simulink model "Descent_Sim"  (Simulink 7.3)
settings: Solver=ode45  StartTime=0.0  StopTime=900  RelTol=1e-3
InitFcn:
  | init
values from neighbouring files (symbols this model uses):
  h0 = 76068    [init.m]
  mass = 450    [init.m]
  sp = 30.81    [init.m]
  x0 = 0    [init.m]
  x_cg = 31.56    [init.m]
  x_ref = 31.5    [init.m]
  y_cg = 0    [init.m]
  z_cg = 1.24    [init.m]
undefined symbols (not defined in the file or in its folder): Altitude2, Cl, Cld1, Cld2, Cld3, Cld4, Cm, Cmd1, Cmd2, Cmd3, Cmd4, Cn, Cnd1, Cnd2, Cnd3, Cnd4, Continuous, CX, CXd1, CXd2, CXd3, CXd4, CY, CYd1, CYd2, CYd3, CYd4, CZ, CZd1, CZd2, CZd3, CZd4, Dryden, F, FCS, ft, km, Light, MIL, q, r, sigbuilder_block, Surf_mix
libraries: aerolibasang x3, aerolibwind2 x3, aerolib6dof2 x1, aerolibconvert2 x1, aerolibatmos2 x1, aerolibgravity2 x1, aerolibadyn x1

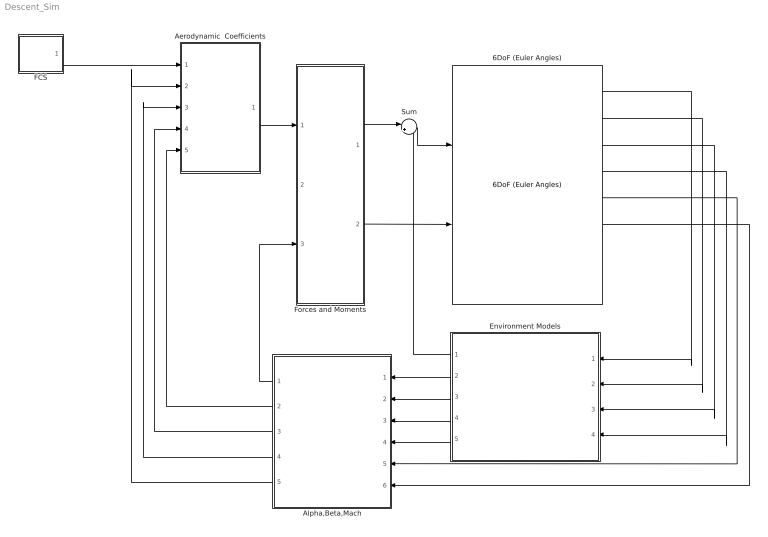
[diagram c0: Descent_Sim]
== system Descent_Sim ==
  6DoF (Euler Angles) : aerolib6dof2/6DoF (Euler Angles)  SystemSampleTime=-1  units=English (Velocity in ft/s)  mtype=Fixed  rep=Euler Angles  xme_0=[-x0, 0, -h0]  Vm_0=Uvw_0  eul_0=Euler_0  pm_0=pqr_0  mass_0=mass  mass_e=0.5  mass_f=2.0  inertia=inertia  inertia_e=eye(3)  inertia_f=2*eye(3)  k_quat=1.0
  Aerodynamic  Coefficients : Subsystem
  Alpha,Beta,Mach : Subsystem
  Environment Models : Subsystem
  FCS : Subsystem
  Forces and Moments : Subsystem
  Sum : Sum  Inputs=|++  OutDataType=sfix(16)  OutScaling=2^0
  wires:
  6DoF (Euler Angles)/5 -> Alpha,Beta,Mach/5(Vb)
  6DoF (Euler Angles)/1 -> Environment Models/1(Ve)
  6DoF (Euler Angles)/2 -> Environment Models/2(Xe)
  6DoF (Euler Angles)/3 -> Environment Models/3(Euler)
  6DoF (Euler Angles)/4 -> Environment Models/4(DCM)
  Sum/1 -> 6DoF (Euler Angles)/1
  Forces and Moments/1(X,Y,Z) -> Sum/1
  Environment Models/2(Speed of Sound) -> Alpha,Beta,Mach/1(Speed of Sound)
  Environment Models/3(Wind Velocity) -> Alpha,Beta,Mach/2(Wind Velocity)
  Environment Models/4(Air Density) -> Alpha,Beta,Mach/3(Air Density)
  Environment Models/5(Wind Angular Rates) -> Alpha,Beta,Mach/4(Wind Angular Rates)
  Environment Models/1(Fg) -> Sum/2
  Alpha,Beta,Mach/1(qbar) -> Forces and Moments/3(qbar)
  Alpha,Beta,Mach/3(V) -> Aerodynamic  Coefficients/4(V)
  Alpha,Beta,Mach/5(Incid) -> Aerodynamic  Coefficients/2(Incid)
  Alpha,Beta,Mach/4(Mach) -> Aerodynamic  Coefficients/3(Mach)
  Alpha,Beta,Mach/2("p,q,r ") -> Aerodynamic  Coefficients/5(p,q,r)
  6DoF (Euler Angles)/6 -> Alpha,Beta,Mach/6(p,q,r)
  Aerodynamic  Coefficients/1(Coeff) -> Forces and Moments/1(Coeff)
  Forces and Moments/2(LMN) -> 6DoF (Euler Angles)/2
  FCS/1(delta) -> Aerodynamic  Coefficients/1(deltas)

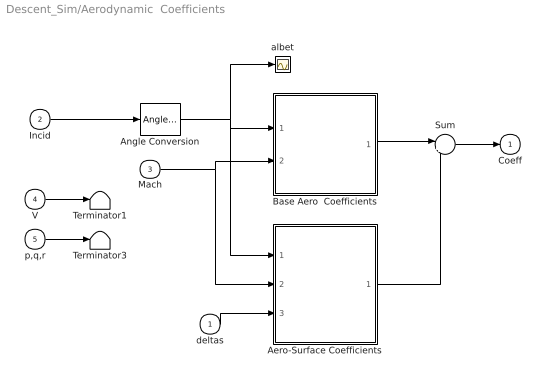
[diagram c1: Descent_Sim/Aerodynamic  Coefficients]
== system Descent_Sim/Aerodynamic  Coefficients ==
  deltas : Inport  OutDataType=sfix(16)  OutScaling=2^0
  Incid : Inport  Port=2  OutDataType=sfix(16)  OutScaling=2^0
  Mach : Inport  Port=3  OutDataType=sfix(16)  OutScaling=2^0
  V : Inport  Port=4  OutDataType=sfix(16)  OutScaling=2^0
  p,q,r : Inport  Port=5  OutDataType=sfix(16)  OutScaling=2^0
  Aero-Surface Coefficients : Subsystem
  Angle Conversion : aerolibconvert2/Angle Conversion  SystemSampleTime=-1  IU=rad  OU=deg
  Base Aero  Coefficients : Subsystem
  Sum : Sum  Inputs=|++  OutDataType=fixdt(1, 16)  OutScaling=2^0
  Terminator1 : Terminator
  Terminator3 : Terminator
  albet : Scope
  Coeff : Outport  OutDataType=sfix(16)  OutScaling=2^0  InitialOutput=0
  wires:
  p,q,r/1 -> Terminator3/1
  V/1 -> Terminator1/1
  Incid/1 -> Angle Conversion/1
  Angle Conversion/1 -> albet/1, Base Aero  Coefficients/1(albet), Aero-Surface Coefficients/1(albet)
  Mach/1 -> Base Aero  Coefficients/2(Mach), Aero-Surface Coefficients/2(Mach)
  Sum/1 -> Coeff/1
  Base Aero  Coefficients/1(Coeff) -> Sum/1
  Aero-Surface Coefficients/1(Coeff) -> Sum/2
  deltas/1 -> Aero-Surface Coefficients/3(delta)

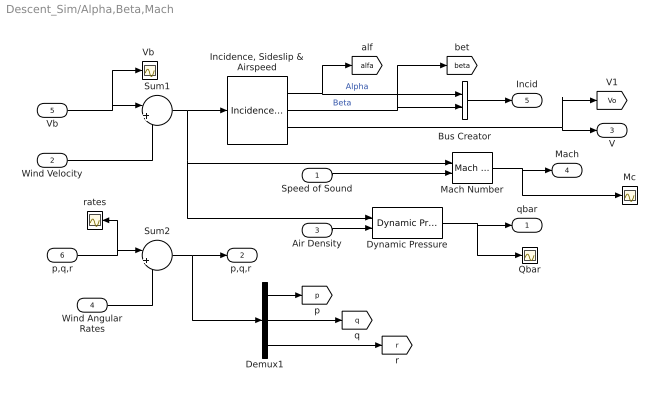
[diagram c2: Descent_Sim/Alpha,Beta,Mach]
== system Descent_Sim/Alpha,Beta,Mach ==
  Speed of Sound : Inport  OutDataType=sfix(16)  OutScaling=2^0
  Wind Velocity : Inport  Port=2  PortDimensions=3  OutDataType=sfix(16)  OutScaling=2^0
  Air Density : Inport  Port=3  OutDataType=sfix(16)  OutScaling=2^0
  Wind Angular Rates : Inport  Port=4  PortDimensions=3  OutDataType=sfix(16)  OutScaling=2^0
  Vb : Inport  Port=5  PortDimensions=3  OutDataType=sfix(16)  OutScaling=2^0
  p,q,r : Inport  Port=6  PortDimensions=3  OutDataType=sfix(16)  OutScaling=2^0
  Bus Creator : BusCreator  Inputs=2
  Demux1 : Demux  Outputs=3
  Dynamic Pressure : aerolibasang/Dynamic Pressure  SystemSampleTime=-1
  "Incidence, Sideslip & Airspeed" : aerolibasang/Incidence, Sideslip, & Airspeed  SystemSampleTime=-1
  Mach Number : aerolibasang/Mach Number  SystemSampleTime=-1
  Mc : Scope
  Qbar : Scope
  Sum1 : Sum  Inputs=|+-  OutDataType=sfix(16)  OutScaling=2^0
  Sum2 : Sum  Inputs=|++  OutDataType=sfix(16)  OutScaling=2^0
  "Vb " : Scope
  rates : Scope
  qbar : Outport  OutDataType=sfix(16)  OutScaling=2^0  InitialOutput=0
  "p,q,r " : Outport  Port=2  OutDataType=sfix(16)  OutScaling=2^0
  V : Outport  Port=3  OutDataType=sfix(16)  OutScaling=2^0
  Mach : Outport  Port=4  OutDataType=sfix(16)  OutScaling=2^0
  Incid : Outport  Port=5  OutDataType=sfix(16)  OutScaling=2^0
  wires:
  "Incidence, Sideslip & Airspeed"/3 -> V/1, [Vo]
  Dynamic Pressure/1 -> qbar/1, Qbar/1
  Air Density/1 -> Dynamic Pressure/2
  Mach Number/1 -> Mach/1, Mc/1
  Sum1/1 -> Dynamic Pressure/1, Mach Number/1, "Incidence, Sideslip & Airspeed"/1
  Vb/1 -> Sum1/1, "Vb "/1
  Speed of Sound/1 -> Mach Number/2
  Wind Velocity/1 -> Sum1/2
  "Incidence, Sideslip & Airspeed"/2 -> Bus Creator/2, [beta]  "Beta"
  Bus Creator/1 -> Incid/1
  "Incidence, Sideslip & Airspeed"/1 -> Bus Creator/1, [alfa]  "Alpha"
  p,q,r/1 -> Sum2/1, rates/1
  Wind Angular Rates/1 -> Sum2/2
  Sum2/1 -> "p,q,r "/1, Demux1/1
  Demux1/2 -> [q]
  Demux1/3 -> [r]
  Demux1/1 -> [p]

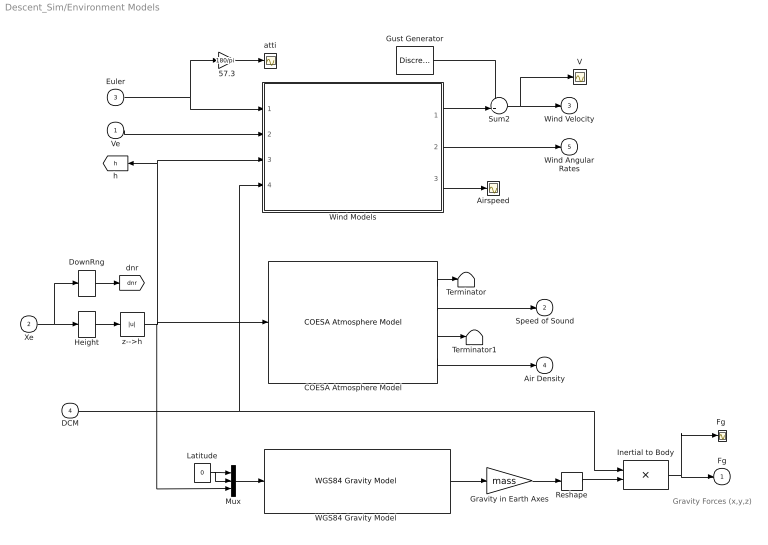
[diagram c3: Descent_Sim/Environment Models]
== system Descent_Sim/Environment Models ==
  note: Gravity Forces (x,y,z)
  Ve : Inport  OutDataType=sfix(16)  OutScaling=2^0
  Xe : Inport  Port=2  PortDimensions=3  OutDataType=sfix(16)  OutScaling=2^0
  Euler : Inport  Port=3  OutDataType=sfix(16)  OutScaling=2^0
  DCM : Inport  Port=4  OutDataType=sfix(16)  OutScaling=2^0
  57.3 : Gain  Gain=180/pi  ParameterDataType=sfix(16)  ParameterScaling=2^0  OutDataType=sfix(16)  OutScaling=2^0
  Airspeed : Scope
  COESA Atmosphere Model : aerolibatmos2/COESA Atmosphere Model  SystemSampleTime=-1  units=English (Velocity in ft/s)  spec=1976 COESA-extended U.S. Standard Atmosphere  model=Profile  profile_var=High temperature  profile_percent=1%  profile_alt=5 km (16404 ft)  envelope_var=High temperature  envelope_percent=1%  action=Warning
  DownRng : Selector  InputPortWidth=3  IndexOptions=Index vector (dialog)  Indices=[1]  OutputSizes=1
  "Fg " : Scope
  Gravity in Earth Axes : Gain  Gain=mass  ParameterDataType=sfix(16)  ParameterScaling=2^0  OutDataType=sfix(16)  OutScaling=2^0
  Gust Generator : DiscretePulseGenerator  PulseType=Time based  Amplitude=[0, 0, 0]  Period=[100, 100, 100]  PulseWidth=1  PhaseDelay=0  SampleTime=1
  Height : Selector  InputPortWidth=3  IndexOptions=Index vector (dialog)  Indices=[3]  OutputSizes=1
  Inertial to Body : Product  Multiplication=Matrix(*)  OutDataType=sfix(16)  OutScaling=2^0
  Latitude : Constant  Value=0  OutDataType=sfix(16)  OutScaling=2^0
  Mux : Mux  Inputs=3
  Reshape : Reshape
  Sum2 : Sum  Inputs=++|  OutDataType=sfix(16)  OutScaling=2^0
  Terminator : Terminator
  Terminator1 : Terminator
  V : Scope
  "WGS84 Gravity Model " : aerolibgravity2/WGS84 Gravity Model   SystemSampleTime=-1  model=WGS84 Taylor Series  units=English  no_atmos=on  precessing=on  jd_loc=off  month=October  day=10  year=2004  no_centrifugal=on  action=None
  Wind Models : Subsystem
  atti : Scope
  z-->h : Abs
  Fg : Outport  OutDataType=sfix(16)  OutScaling=2^0  InitialOutput=0
  Speed of Sound : Outport  Port=2  OutDataType=sfix(16)  OutScaling=2^0  InitialOutput=0
  Wind Velocity : Outport  Port=3  OutDataType=sfix(16)  OutScaling=2^0  InitialOutput=0
  Air Density : Outport  Port=4  OutDataType=sfix(16)  OutScaling=2^0  InitialOutput=0
  Wind Angular Rates : Outport  Port=5  OutDataType=sfix(16)  OutScaling=2^0  InitialOutput=0
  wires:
  Reshape/1 -> Inertial to Body/2
  "WGS84 Gravity Model "/1 -> Gravity in Earth Axes/1
  Gravity in Earth Axes/1 -> Reshape/1
  COESA Atmosphere Model/1 -> Terminator/1
  COESA Atmosphere Model/2 -> Speed of Sound/1
  COESA Atmosphere Model/3 -> Terminator1/1
  COESA Atmosphere Model/4 -> Air Density/1
  DCM/1 -> Inertial to Body/1, Wind Models/4(DCM)
  Inertial to Body/1 -> Fg/1, "Fg "/1
  Mux/1 -> "WGS84 Gravity Model "/1
  Latitude/1 -> Mux/2, Mux/1
  Height/1 -> z-->h/1
  Xe/1 -> Height/1, DownRng/1
  z-->h/1 -> COESA Atmosphere Model/1, Mux/3, Wind Models/3(Altitude), [h]
  Euler/1 -> Wind Models/1(Euler), 57.3/1
  Wind Models/2(pg,qg,rg) -> Wind Angular Rates/1
  Wind Models/3(Airspeed) -> Airspeed/1
  Ve/1 -> Wind Models/2(Ve)
  Sum2/1 -> Wind Velocity/1, V/1
  Wind Models/1(ug,vg,wg) -> Sum2/2
  Gust Generator/1 -> Sum2/1
  DownRng/1 -> [dnr]
  57.3/1 -> atti/1

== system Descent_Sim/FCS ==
  note: Control Surface Mixing Logic Matrix from FCS Demands
  Aero Surface  Mixing Logic : Subsystem
  Bus Creator1 : BusCreator  Inputs='Elevon','Body-Flap','Aileron','Rudder'
  Demux : Demux
  Flight Control System : Subsystem
  "delta " : Scope
  delta : Outport
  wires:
  Bus Creator1/1 -> delta/1
  Demux/1 -> Bus Creator1/1  "Elevon"
  Demux/2 -> Bus Creator1/2  "Body-Flap"
  Demux/3 -> Bus Creator1/3  "Aileron"
  Flight Control System/1(FCS dem) -> Aero Surface  Mixing Logic/1(DPQR)
  Aero Surface  Mixing Logic/1(delta) -> "delta "/1, Demux/1
  Demux/4 -> Bus Creator1/4  "Rudder"

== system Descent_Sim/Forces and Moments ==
  note: Aero coefficients (CX,CY,CZ,Cl,Cm,Cn)
  note: Dynamic Pressure
  Coeff : Inport  OutDataType=sfix(16)  OutScaling=2^0
  Thrust : Inport  Port=2  OutDataType=sfix(16)  OutScaling=2^0
  qbar : Inport  Port=3  OutDataType=sfix(16)  OutScaling=2^0
  "Aerodynamic Forces and Moments (Fx,Fy,Fz), (Lx,My,Nz)" : aerolibadyn/Aerodynamic Forces and Moments   SystemSampleTime=-1  inputAxes=Body  outputForceAxes=Body  outputMomentAxes=Body  S=Sref  b=sp  cbar=ch
  CG : Step  Time=250*[1 1 1]  Before="[x_cg, y_cg,  z_cg]"  After="[x_cg,  y_cg+0.3,  z_cg]"
  Center of Gravity : Constant  Value=[x_cg, y_cg, z_cg]  OutDataType=sfix(16)  OutScaling=2^0
  "Force " : Scope
  Force ---> Acc : Gain  Gain=1/mass  ParameterDataType=sfix(16)  ParameterScaling=2^0  OutDataType=sfix(16)  OutScaling=2^0
  Moments : Scope
  Moments Reference Center (MRC) in (feet) : Constant  Value=[x_ref 0 0]  OutDataType=sfix(16)  OutScaling=2^0
  Sum1 : Sum  Inputs=++|  OutDataType=sfix(16)  OutScaling=2^0
  X,Y,Z : Outport  OutDataType=sfix(16)  OutScaling=2^0  InitialOutput=0
  LMN : Outport  Port=2  OutDataType=sfix(16)  OutScaling=2^0  InitialOutput=0
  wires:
  Coeff/1 -> "Aerodynamic Forces and Moments (Fx,Fy,Fz), (Lx,My,Nz)"/1
  qbar/1 -> "Aerodynamic Forces and Moments (Fx,Fy,Fz), (Lx,My,Nz)"/2
  Thrust/1 -> Sum1/1
  Sum1/1 -> Force ---> Acc/1, X,Y,Z/1, "Force "/1
  "Aerodynamic Forces and Moments (Fx,Fy,Fz), (Lx,My,Nz)"/1 -> Sum1/2
  Moments Reference Center (MRC) in (feet)/1 -> "Aerodynamic Forces and Moments (Fx,Fy,Fz), (Lx,My,Nz)"/4
  "Aerodynamic Forces and Moments (Fx,Fy,Fz), (Lx,My,Nz)"/2 -> LMN/1, Moments/1
  Center of Gravity/1 -> "Aerodynamic Forces and Moments (Fx,Fy,Fz), (Lx,My,Nz)"/3

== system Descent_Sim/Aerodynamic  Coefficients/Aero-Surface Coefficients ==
  note: Surface Coefficients
  albet : Inport
  Mach : Inport  Port=2
  delta : Inport  Port=3
  Aileron : Subsystem
  Body-Flap : Subsystem
  Elevon : Subsystem
  Rudder : Subsystem
  Sum : Sum  Inputs=++++  OutDataType=fixdt(1, 16)  OutScaling=2^0
  Coeff : Outport
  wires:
  Elevon/1(Coeff) -> Sum/1
  delta/1 -> Elevon/3(delta), Body-Flap/3(delta), Aileron/3(delta), Rudder/3(delta)
  Body-Flap/1(Coeff) -> Sum/2
  Rudder/1(Coeff) -> Sum/4
  albet/1 -> Elevon/1(albet), Body-Flap/1(albet), Aileron/1(albet), Rudder/1(albet)
  Mach/1 -> Elevon/2(Mach), Body-Flap/2(Mach), Aileron/2(Mach), Rudder/2(Mach)
  Aileron/1(Coeff) -> Sum/3
  Sum/1 -> Coeff/1

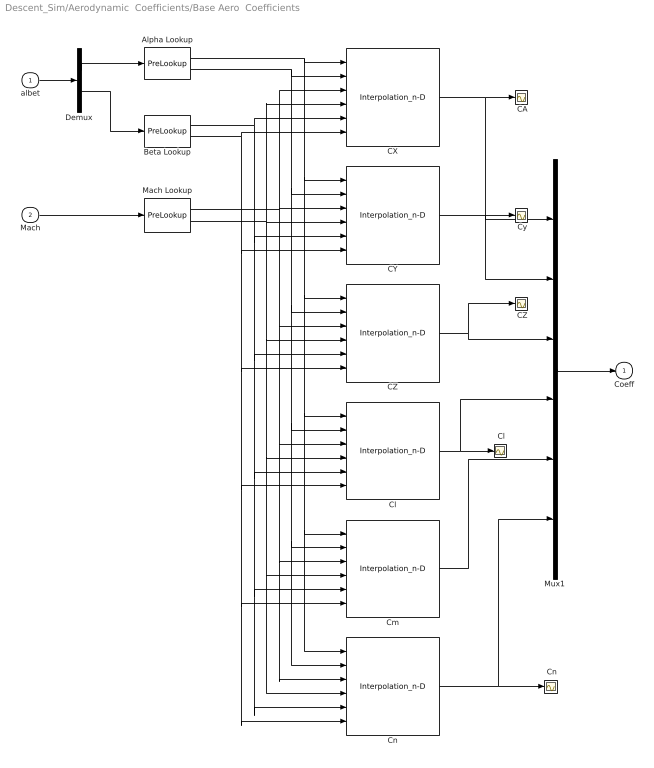
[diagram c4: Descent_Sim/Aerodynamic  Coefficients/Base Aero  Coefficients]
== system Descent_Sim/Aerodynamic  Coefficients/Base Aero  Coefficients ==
  albet : Inport  OutDataType=sfix(16)  OutScaling=2^0
  Mach : Inport  Port=2  OutDataType=sfix(16)  OutScaling=2^0
  " CA" : Scope
  " CZ" : Scope
  " Cl" : Scope
  " Cn" : Scope
  " Cy" : Scope
  Alpha Lookup : PreLookup  BreakpointsData=Alfas  BeginIndexSearchUsingPreviousIndexResult=on  ProcessOutOfRangeInput=Linear extrapolation  IndexDataType=sfix(16)  FractionDataType=sfix(16)  FractionScaling=2^0
  Beta Lookup : PreLookup  BreakpointsData=Betas  BeginIndexSearchUsingPreviousIndexResult=on  ProcessOutOfRangeInput=Linear extrapolation  IndexDataType=sfix(16)  FractionDataType=sfix(16)  FractionScaling=2^0
  CX : Interpolation_n-D  NumberOfTableDimensions=3  Table=CX  CheckIndexInCode=off  OutDataType=sfix(16)  OutScaling=2^0
  CY : Interpolation_n-D  NumberOfTableDimensions=3  Table=CY  CheckIndexInCode=off  OutDataType=sfix(16)  OutScaling=2^0
  CZ : Interpolation_n-D  NumberOfTableDimensions=3  Table=CZ  CheckIndexInCode=off  OutDataType=sfix(16)  OutScaling=2^0
  Cl : Interpolation_n-D  NumberOfTableDimensions=3  Table=Cl  CheckIndexInCode=off  OutDataTypeMode=double  OutDataType=sfix(16)  OutScaling=2^0  OutDataTypeStr=double
  Cm : Interpolation_n-D  NumberOfTableDimensions=3  Table=Cm  CheckIndexInCode=off  OutDataType=sfix(16)  OutScaling=2^0
  Cn : Interpolation_n-D  NumberOfTableDimensions=3  Table=Cn  CheckIndexInCode=off  OutDataType=sfix(16)  OutScaling=2^0
  Demux : Demux  Outputs=2
  Mach Lookup : PreLookup  BreakpointsData=Machs  BeginIndexSearchUsingPreviousIndexResult=on  ProcessOutOfRangeInput=Linear extrapolation  IndexDataType=sfix(16)  FractionDataType=sfix(16)  FractionScaling=2^0
  Mux1 : Mux  Inputs=6
  Coeff : Outport  OutDataType=sfix(16)  OutScaling=2^0  InitialOutput=0
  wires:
  Demux/1 -> Alpha Lookup/1
  CX/1 -> Mux1/1, " CA"/1
  CY/1 -> Mux1/2, " Cy"/1
  CZ/1 -> Mux1/3, " CZ"/1
  Cl/1 -> Mux1/4, " Cl"/1
  Cm/1 -> Mux1/5
  Cn/1 -> Mux1/6, " Cn"/1
  Alpha Lookup/1 -> CX/1, CY/1, Cm/1, Cn/1, Cl/1, CZ/1
  Alpha Lookup/2 -> CX/2, CY/2, CZ/2, Cl/2, Cm/2, Cn/2
  Mach Lookup/1 -> CY/3, Cm/3, Cn/3, Cl/3, CZ/3, CX/3
  Mach Lookup/2 -> CY/4, Cm/4, Cn/4, Cl/4, CZ/4, CX/4
  Beta Lookup/1 -> CX/5, Cm/5, Cn/5, Cl/5, CZ/5, CY/5
  Beta Lookup/2 -> CX/6, CY/6, Cm/6, Cn/6, Cl/6, CZ/6
  Mux1/1 -> Coeff/1
  Demux/2 -> Beta Lookup/1
  albet/1 -> Demux/1
  Mach/1 -> Mach Lookup/1

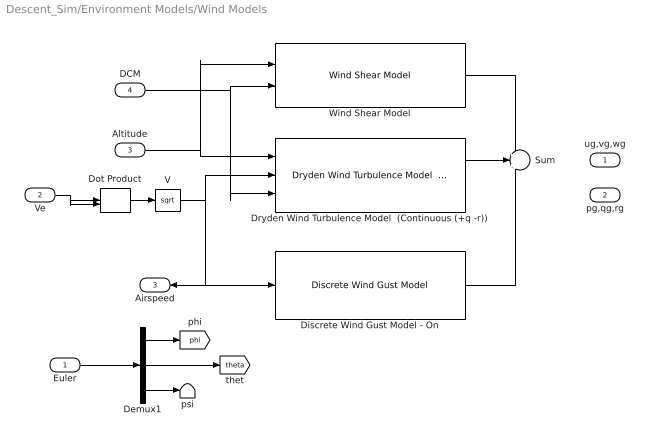
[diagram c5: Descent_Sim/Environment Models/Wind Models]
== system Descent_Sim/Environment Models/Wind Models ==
  Euler : Inport  OutDataType=sfix(16)  OutScaling=2^0
  Ve : Inport  Port=2  OutDataType=sfix(16)  OutScaling=2^0
  Altitude : Inport  Port=3  OutDataType=sfix(16)  OutScaling=2^0
  DCM : Inport  Port=4  OutDataType=sfix(16)  OutScaling=2^0
  Demux1 : Demux  Outputs=3
  Discrete Wind Gust Model - On : aerolibwind2/Discrete Wind Gust Model  SystemSampleTime=-1  units=English (Velocity in ft/s)  Gx=on  Gy=on  Gz=on  t_0=20  d_m=[120 120 80]  v_m=[3.5 3.0 3.0]
  Dot Product : DotProduct  OutDataType=sfix(16)  OutScaling=2^-10  SaturateOnIntegerOverflow=on
  Dryden Wind Turbulence Model  (Continuous (+q -r)) : aerolibwind2/Dryden Wind Turbulence Model  (Continuous (+q -r))  SystemSampleTime=-1  units=English (Velocity in ft/s)  spec=MIL-F-8785C  model=Continuous Dryden (+q -r)  W20=5  Wdeg=0  TurbProb=10^-2 - Light  L_high=533.4  Wingspan=4  ts=0.1  Seed=[23341 23342 23343 23344]  T_on=on
  Sum : Sum  Inputs=+++  OutDataType=sfix(16)  OutScaling=2^0
  V : Math  Operator=sqrt  OutDataType=sfix(16)  OutScaling=2^0
  Wind Shear Model : aerolibwind2/Wind Shear Model  SystemSampleTime=-1  units=English (Velocity in ft/s)  phase=Category C - Terminal Flight Phase  W_20=1  Wdeg=0
  psi : Terminator
  ug,vg,wg : Outport  OutDataType=sfix(16)  OutScaling=2^0
  pg,qg,rg : Outport  Port=2  OutDataType=sfix(16)  OutScaling=2^0
  Airspeed : Outport  Port=3  OutDataType=sfix(16)  OutScaling=2^0
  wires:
  Dryden Wind Turbulence Model  (Continuous (+q -r))/1 -> Sum/2
  Discrete Wind Gust Model - On/1 -> Sum/3
  Wind Shear Model/1 -> Sum/1
  DCM/1 -> Wind Shear Model/2, Dryden Wind Turbulence Model  (Continuous (+q -r))/3
  Altitude/1 -> Dryden Wind Turbulence Model  (Continuous (+q -r))/1, Wind Shear Model/1
  Euler/1 -> Demux1/1
  Dot Product/1 -> V/1
  Ve/1 -> Dot Product/1, Dot Product/2
  V/1 -> Dryden Wind Turbulence Model  (Continuous (+q -r))/2, Discrete Wind Gust Model - On/1, Airspeed/1
  Demux1/2 -> [theta]
  Demux1/1 -> [phi]
  Demux1/3 -> psi/1

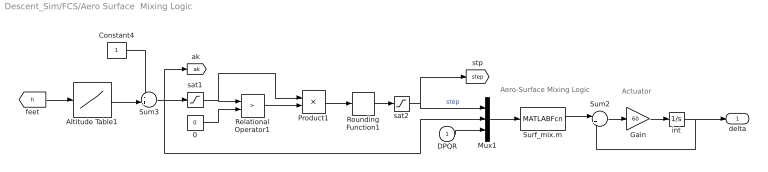
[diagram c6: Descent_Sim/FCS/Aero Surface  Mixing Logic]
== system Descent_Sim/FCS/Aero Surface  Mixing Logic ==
  note: Aero-Surface Mixing Logic
  note: Actuator
  DPQR : Inport  OutDataType=sfix(16)  OutScaling=2^0
  0 : Constant  Value=0  OutDataType=fixdt(1, 16)  OutScaling=2^0
  Altitude Table1 : Lookup  InputValues=Altitude2(:,1)  Table=Altitude2(:,2)  OutDataType=fixdt(1, 16)  OutScaling=2^0
  Constant4 : Constant  OutDataType=fixdt(1, 16)  OutScaling=2^0
  Gain : Gain  Gain=60  ParameterDataType=fixdt(1, 16)  ParameterScaling=2^0  OutDataType=fixdt(1, 16)  OutScaling=2^0
  Mux1 : Mux  Inputs=[1, 1, 3]
  Product1 : Product  OutDataType=fixdt(1, 16)  OutScaling=2^0
  Relational Operator1 : RelationalOperator  Operator=>  LogicOutDataTypeMode=boolean  LogicDataType=fixdt(0, 8)  OutDataTypeStr=boolean
  Rounding Function1 : Rounding  Operator=ceil
  Sum2 : Sum  Inputs=|+-  OutDataType=fixdt(1, 16)  OutScaling=2^0
  Sum3 : Sum  Inputs=-+|  OutDataType=fixdt(1, 16)  OutScaling=2^0
  Surf_mix.m : MATLABFcn  MATLABFcn=Surf_mix(u(1), u(2), u(3:5) )  OutputDimensions=4
  int : Integrator  InitialCondition=[0.08, 0.02, 0, 0]
  sat1 : Saturate  UpperLimit=12  LowerLimit=1  OutDataType=fixdt(1, 16)  OutScaling=2^0
  sat2 : Saturate  UpperLimit=12  LowerLimit=1  OutDataType=fixdt(1, 16)  OutScaling=2^0
  delta : Outport
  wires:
  [h] -> Altitude Table1/1
  0/1 -> Relational Operator1/2
  Relational Operator1/1 -> Product1/2
  Product1/1 -> Rounding Function1/1
  Rounding Function1/1 -> sat2/1
  sat1/1 -> Relational Operator1/1, Product1/1
  Constant4/1 -> Sum3/1
  Altitude Table1/1 -> Sum3/2
  Sum3/1 -> sat1/1, Mux1/2, [ak]
  sat2/1 -> Mux1/1, [step]  "step"
  Mux1/1 -> Surf_mix.m/1
  Surf_mix.m/1 -> Sum2/1
  DPQR/1 -> Mux1/3
  Gain/1 -> int/1
  Sum2/1 -> Gain/1
  int/1 -> Sum2/2, delta/1

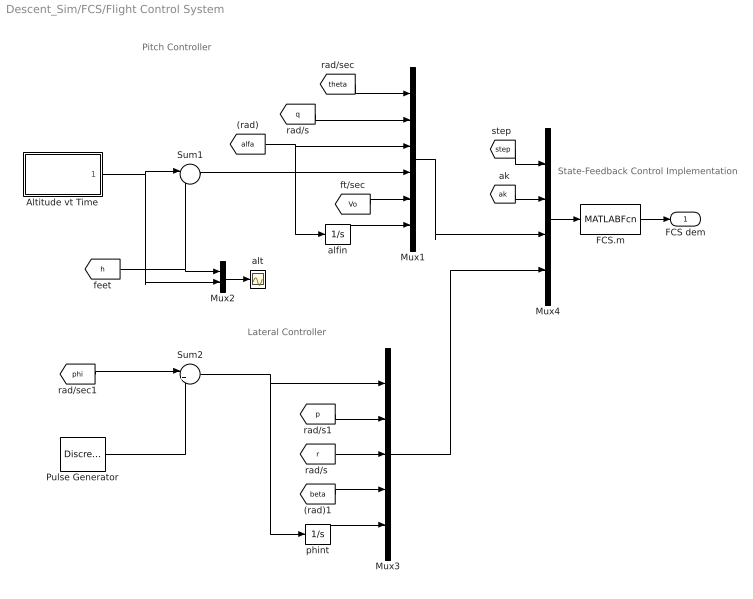
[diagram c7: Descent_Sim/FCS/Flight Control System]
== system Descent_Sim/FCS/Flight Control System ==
  note: Pitch Controller
  note: Lateral Controller
  note: State-Feedback Control Implementation
  Altitude vt Time : Subsystem  Tag=STV Subsys  LoadFcn=sigbuilder_block('load');  StartFcn=sigbuilder_block('start');  StopFcn=sigbuilder_block('stop');  ClipboardFcn=sigbuilder_block('clipboard');
  FCS.m : MATLABFcn  MATLABFcn=FCS(u(1), u(2), u(3:8), u(9:13) )  OutputDimensions=3
  Mux1 : Mux  Inputs=6
  Mux2 : Mux  Inputs=2
  Mux3 : Mux  Inputs=5
  Mux4 : Mux  Inputs=[1, 1, 6, 5]
  Pulse Generator : DiscretePulseGenerator  PulseType=Time based  Amplitude=0*(pi/180)  Period=500  PulseWidth=5  PhaseDelay=40  SampleTime=1
  Sum1 : Sum  Inputs=|-+  OutDataType=fixdt(1, 16)  OutScaling=2^0
  Sum2 : Sum  Inputs=|+-  OutDataType=fixdt(1, 16)  OutScaling=2^0
  alfin : Integrator
  alt : Scope
  phint : Integrator
  FCS dem : Outport
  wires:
  alfin/1 -> Mux1/6
  [q] -> Mux1/2
  [theta] -> Mux1/1
  [alfa] -> Mux1/3, alfin/1
  [h] -> Sum1/2, Mux2/1
  Sum1/1 -> Mux1/4
  [p] -> Mux3/2
  [r] -> Mux3/3
  Sum2/1 -> Mux3/1, phint/1
  FCS.m/1 -> FCS dem/1
  Mux1/1 -> Mux4/3
  [Vo] -> Mux1/5
  Mux2/1 -> alt/1
  [beta] -> Mux3/4
  phint/1 -> Mux3/5
  Mux3/1 -> Mux4/4
  Altitude vt Time/1(Signal 1) -> Sum1/1, Mux2/2
  Mux4/1 -> FCS.m/1
  [step] -> Mux4/1
  [ak] -> Mux4/2
  [phi] -> Sum2/1
  Pulse Generator/1 -> Sum2/2

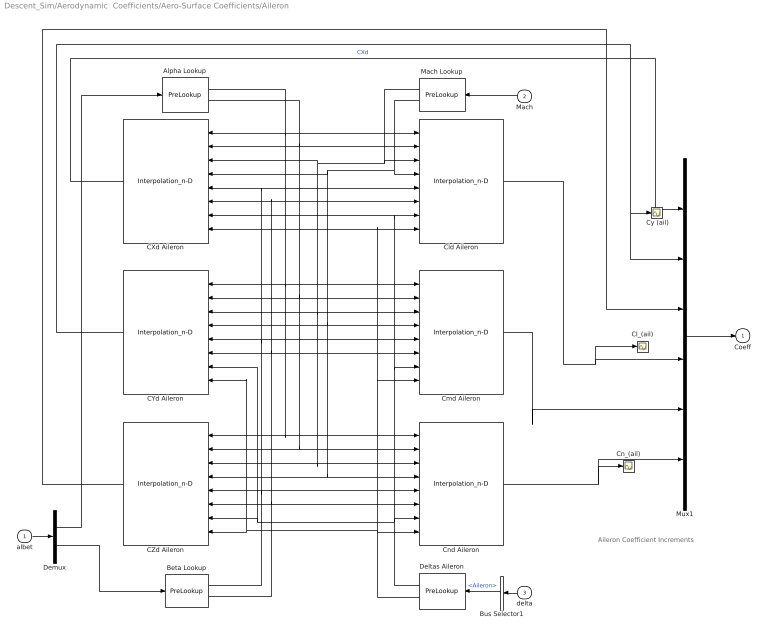
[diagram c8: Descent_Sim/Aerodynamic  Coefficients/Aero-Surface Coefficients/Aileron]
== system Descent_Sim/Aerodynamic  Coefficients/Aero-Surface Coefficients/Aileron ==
  note: Aileron Coefficient Increments
  albet : Inport  OutDataType=sfix(16)  OutScaling=2^0
  Mach : Inport  Port=2  OutDataType=sfix(16)  OutScaling=2^0
  delta : Inport  Port=3  OutDataType=sfix(16)  OutScaling=2^0
  " Cy (ail)" : Scope
  Alpha Lookup : PreLookup  BreakpointsData=Alfas  BeginIndexSearchUsingPreviousIndexResult=on  ProcessOutOfRangeInput=Linear extrapolation  IndexDataType=sfix(16)  FractionDataType=sfix(16)  FractionScaling=2^0
  Beta Lookup : PreLookup  BreakpointsData=Betas  BeginIndexSearchUsingPreviousIndexResult=on  ProcessOutOfRangeInput=Linear extrapolation  IndexDataType=sfix(16)  FractionDataType=sfix(16)  FractionScaling=2^0
  Bus Selector1 : BusSelector  OutputSignals=Aileron
  CXd Aileron : Interpolation_n-D  NumberOfTableDimensions=4  Table=CXd3  CheckIndexInCode=off  OutDataType=sfix(16)  OutScaling=2^0
  CYd Aileron : Interpolation_n-D  NumberOfTableDimensions=4  Table=CYd3  CheckIndexInCode=off  OutDataType=sfix(16)  OutScaling=2^0
  CZd Aileron : Interpolation_n-D  NumberOfTableDimensions=4  Table=CZd3  CheckIndexInCode=off  OutDataType=sfix(16)  OutScaling=2^0
  Cl_(ail) : Scope
  Cld Aileron : Interpolation_n-D  NumberOfTableDimensions=4  Table=Cld3  CheckIndexInCode=off  OutDataType=sfix(16)  OutScaling=2^0
  Cmd Aileron : Interpolation_n-D  NumberOfTableDimensions=4  Table=Cmd3  CheckIndexInCode=off  OutDataType=sfix(16)  OutScaling=2^0
  Cn_(ail) : Scope
  Cnd Aileron : Interpolation_n-D  NumberOfTableDimensions=4  Table=Cnd3  CheckIndexInCode=off  OutDataType=sfix(16)  OutScaling=2^0
  Deltas Aileron : PreLookup  BreakpointsData=Deltas3  BeginIndexSearchUsingPreviousIndexResult=on  ProcessOutOfRangeInput=Linear extrapolation  IndexDataType=sfix(16)  FractionDataType=sfix(16)  FractionScaling=2^0
  Demux : Demux  Outputs=2
  Mach Lookup : PreLookup  BreakpointsData=Machs  BeginIndexSearchUsingPreviousIndexResult=on  ProcessOutOfRangeInput=Linear extrapolation  IndexDataType=sfix(16)  FractionDataType=sfix(16)  FractionScaling=2^0
  Mux1 : Mux  Inputs=6
  Coeff : Outport  OutDataType=sfix(16)  OutScaling=2^0  InitialOutput=0
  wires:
  CZd Aileron/1 -> Mux1/3
  CYd Aileron/1 -> Mux1/2, " Cy (ail)"/1
  CXd Aileron/1 -> Mux1/1  "CXd"
  delta/1 -> Bus Selector1/1
  Demux/2 -> Beta Lookup/1
  Mach/1 -> Mach Lookup/1
  Demux/1 -> Alpha Lookup/1
  Cld Aileron/1 -> Mux1/4, Cl_(ail)/1
  Cmd Aileron/1 -> Mux1/5
  Cnd Aileron/1 -> Mux1/6, Cn_(ail)/1
  Mux1/1 -> Coeff/1
  Deltas Aileron/2 -> CXd Aileron/8, Cld Aileron/8, Cmd Aileron/8, Cnd Aileron/8, CYd Aileron/8, CZd Aileron/8
  Deltas Aileron/1 -> CXd Aileron/7, Cld Aileron/7, Cmd Aileron/7, Cnd Aileron/7, CYd Aileron/7, CZd Aileron/7
  Beta Lookup/2 -> Cld Aileron/6, CXd Aileron/6, Cmd Aileron/6, CYd Aileron/6, Cnd Aileron/6, CZd Aileron/6
  Beta Lookup/1 -> Cld Aileron/5, CXd Aileron/5, Cmd Aileron/5, CYd Aileron/5, Cnd Aileron/5, CZd Aileron/5
  Mach Lookup/2 -> Cnd Aileron/4, CZd Aileron/4, Cmd Aileron/4, CYd Aileron/4, CXd Aileron/4, Cld Aileron/4
  Mach Lookup/1 -> Cnd Aileron/3, CZd Aileron/3, Cmd Aileron/3, CYd Aileron/3, CXd Aileron/3, Cld Aileron/3
  Alpha Lookup/2 -> Cnd Aileron/2, CZd Aileron/2, Cmd Aileron/2, CYd Aileron/2, Cld Aileron/2, CXd Aileron/2
  Alpha Lookup/1 -> Cnd Aileron/1, CZd Aileron/1, Cmd Aileron/1, CYd Aileron/1, Cld Aileron/1, CXd Aileron/1
  albet/1 -> Demux/1
  Bus Selector1/1 -> Deltas Aileron/1  "<Aileron>"

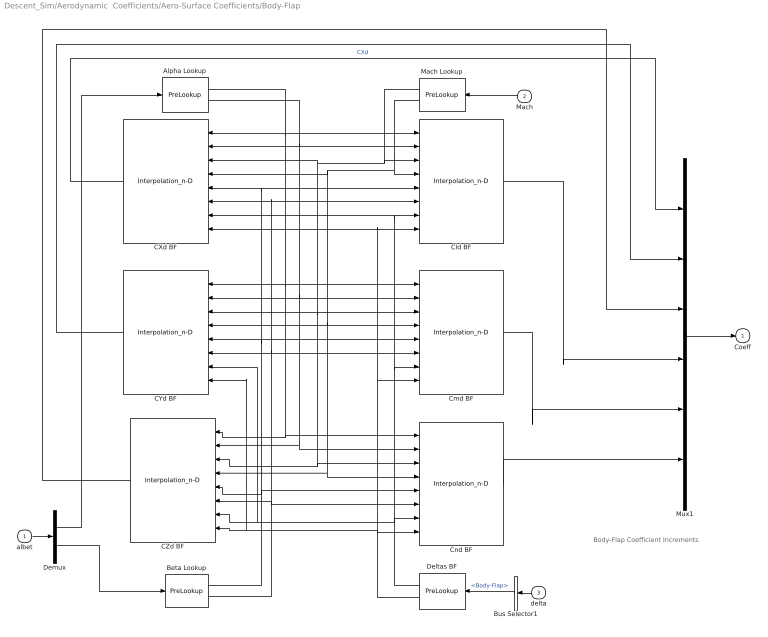
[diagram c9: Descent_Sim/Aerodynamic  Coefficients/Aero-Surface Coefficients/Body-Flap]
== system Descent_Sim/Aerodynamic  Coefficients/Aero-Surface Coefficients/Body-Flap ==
  note: Body-Flap Coefficient Increments
  albet : Inport  OutDataType=sfix(16)  OutScaling=2^0
  Mach : Inport  Port=2  OutDataType=sfix(16)  OutScaling=2^0
  delta : Inport  Port=3  OutDataType=sfix(16)  OutScaling=2^0
  Alpha Lookup : PreLookup  BreakpointsData=Alfas  BeginIndexSearchUsingPreviousIndexResult=on  ProcessOutOfRangeInput=Linear extrapolation  IndexDataType=sfix(16)  FractionDataType=sfix(16)  FractionScaling=2^0
  Beta Lookup : PreLookup  BreakpointsData=Betas  BeginIndexSearchUsingPreviousIndexResult=on  ProcessOutOfRangeInput=Linear extrapolation  IndexDataType=sfix(16)  FractionDataType=sfix(16)  FractionScaling=2^0
  Bus Selector1 : BusSelector  OutputSignals=Body-Flap
  CXd BF : Interpolation_n-D  NumberOfTableDimensions=4  Table=CXd2  CheckIndexInCode=off  OutDataType=sfix(16)  OutScaling=2^0
  CYd BF : Interpolation_n-D  NumberOfTableDimensions=4  Table=CYd2  CheckIndexInCode=off  OutDataType=sfix(16)  OutScaling=2^0
  CZd BF : Interpolation_n-D  NumberOfTableDimensions=4  Table=CZd2  CheckIndexInCode=off  OutDataType=sfix(16)  OutScaling=2^0
  Cld BF : Interpolation_n-D  NumberOfTableDimensions=4  Table=Cld2  CheckIndexInCode=off  OutDataType=sfix(16)  OutScaling=2^0
  Cmd BF : Interpolation_n-D  NumberOfTableDimensions=4  Table=Cmd2  CheckIndexInCode=off  OutDataType=sfix(16)  OutScaling=2^0
  Cnd BF : Interpolation_n-D  NumberOfTableDimensions=4  Table=Cnd2  CheckIndexInCode=off  OutDataType=sfix(16)  OutScaling=2^0
  Deltas BF : PreLookup  BreakpointsData=Deltas2  BeginIndexSearchUsingPreviousIndexResult=on  ProcessOutOfRangeInput=Linear extrapolation  IndexDataType=sfix(16)  FractionDataType=sfix(16)  FractionScaling=2^0
  Demux : Demux  Outputs=2
  Mach Lookup : PreLookup  BreakpointsData=Machs  BeginIndexSearchUsingPreviousIndexResult=on  ProcessOutOfRangeInput=Linear extrapolation  IndexDataType=sfix(16)  FractionDataType=sfix(16)  FractionScaling=2^0
  Mux1 : Mux  Inputs=6
  Coeff : Outport  OutDataType=sfix(16)  OutScaling=2^0  InitialOutput=0
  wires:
  CZd BF/1 -> Mux1/3
  CYd BF/1 -> Mux1/2
  CXd BF/1 -> Mux1/1  "CXd"
  delta/1 -> Bus Selector1/1
  Demux/2 -> Beta Lookup/1
  Mach/1 -> Mach Lookup/1
  Demux/1 -> Alpha Lookup/1
  Cld BF/1 -> Mux1/4
  Cmd BF/1 -> Mux1/5
  Cnd BF/1 -> Mux1/6
  Mux1/1 -> Coeff/1
  Deltas BF/2 -> CXd BF/8, Cld BF/8, Cmd BF/8, Cnd BF/8, CYd BF/8, CZd BF/8
  Deltas BF/1 -> CXd BF/7, Cld BF/7, Cmd BF/7, Cnd BF/7, CYd BF/7, CZd BF/7
  Beta Lookup/2 -> Cld BF/6, CXd BF/6, Cmd BF/6, CYd BF/6, Cnd BF/6, CZd BF/6
  Beta Lookup/1 -> Cld BF/5, CXd BF/5, Cmd BF/5, CYd BF/5, Cnd BF/5, CZd BF/5
  Mach Lookup/2 -> Cnd BF/4, CZd BF/4, Cmd BF/4, CYd BF/4, CXd BF/4, Cld BF/4
  Mach Lookup/1 -> Cnd BF/3, CZd BF/3, Cmd BF/3, CYd BF/3, CXd BF/3, Cld BF/3
  Alpha Lookup/2 -> Cnd BF/2, CZd BF/2, Cmd BF/2, CYd BF/2, Cld BF/2, CXd BF/2
  Alpha Lookup/1 -> Cnd BF/1, CZd BF/1, Cmd BF/1, CYd BF/1, Cld BF/1, CXd BF/1
  albet/1 -> Demux/1
  Bus Selector1/1 -> Deltas BF/1  "<Body-Flap>"

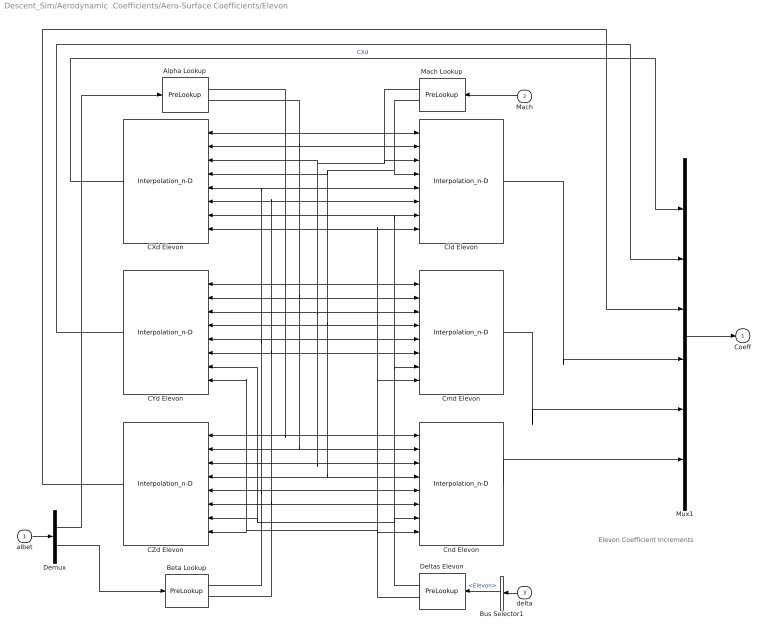
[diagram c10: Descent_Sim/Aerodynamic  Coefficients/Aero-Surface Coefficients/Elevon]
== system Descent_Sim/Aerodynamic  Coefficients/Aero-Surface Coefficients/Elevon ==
  note: Elevon Coefficient Increments
  albet : Inport  OutDataType=sfix(16)  OutScaling=2^0
  Mach : Inport  Port=2  OutDataType=sfix(16)  OutScaling=2^0
  delta : Inport  Port=3  OutDataType=sfix(16)  OutScaling=2^0
  Alpha Lookup : PreLookup  BreakpointsData=Alfas  BeginIndexSearchUsingPreviousIndexResult=on  ProcessOutOfRangeInput=Linear extrapolation  IndexDataType=sfix(16)  FractionDataType=sfix(16)  FractionScaling=2^0
  Beta Lookup : PreLookup  BreakpointsData=Betas  BeginIndexSearchUsingPreviousIndexResult=on  ProcessOutOfRangeInput=Linear extrapolation  IndexDataType=sfix(16)  FractionDataType=sfix(16)  FractionScaling=2^0
  Bus Selector1 : BusSelector  OutputSignals=Elevon
  CXd Elevon : Interpolation_n-D  NumberOfTableDimensions=4  Table=CXd1  CheckIndexInCode=off  OutDataType=sfix(16)  OutScaling=2^0
  CYd Elevon : Interpolation_n-D  NumberOfTableDimensions=4  Table=CYd1  CheckIndexInCode=off  OutDataType=sfix(16)  OutScaling=2^0
  CZd Elevon : Interpolation_n-D  NumberOfTableDimensions=4  Table=CZd1  CheckIndexInCode=off  OutDataType=sfix(16)  OutScaling=2^0
  Cld Elevon : Interpolation_n-D  NumberOfTableDimensions=4  Table=Cld1  CheckIndexInCode=off  OutDataType=sfix(16)  OutScaling=2^0
  Cmd Elevon : Interpolation_n-D  NumberOfTableDimensions=4  Table=Cmd1  CheckIndexInCode=off  OutDataType=sfix(16)  OutScaling=2^0
  Cnd Elevon : Interpolation_n-D  NumberOfTableDimensions=4  Table=Cnd1  CheckIndexInCode=off  OutDataType=sfix(16)  OutScaling=2^0
  Deltas Elevon : PreLookup  BreakpointsData=Deltas1  BeginIndexSearchUsingPreviousIndexResult=on  ProcessOutOfRangeInput=Linear extrapolation  IndexDataType=sfix(16)  FractionDataType=sfix(16)  FractionScaling=2^0
  Demux : Demux  Outputs=2
  Mach Lookup : PreLookup  BreakpointsData=Machs  BeginIndexSearchUsingPreviousIndexResult=on  ProcessOutOfRangeInput=Linear extrapolation  IndexDataType=sfix(16)  FractionDataType=sfix(16)  FractionScaling=2^0
  Mux1 : Mux  Inputs=6
  Coeff : Outport  OutDataType=sfix(16)  OutScaling=2^0  InitialOutput=0
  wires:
  CZd Elevon/1 -> Mux1/3
  CYd Elevon/1 -> Mux1/2
  CXd Elevon/1 -> Mux1/1  "CXd"
  Demux/2 -> Beta Lookup/1
  Mach/1 -> Mach Lookup/1
  Demux/1 -> Alpha Lookup/1
  Cld Elevon/1 -> Mux1/4
  Cmd Elevon/1 -> Mux1/5
  Cnd Elevon/1 -> Mux1/6
  Mux1/1 -> Coeff/1
  Deltas Elevon/2 -> CXd Elevon/8, Cld Elevon/8, Cmd Elevon/8, Cnd Elevon/8, CYd Elevon/8, CZd Elevon/8
  Deltas Elevon/1 -> CXd Elevon/7, Cld Elevon/7, Cmd Elevon/7, Cnd Elevon/7, CYd Elevon/7, CZd Elevon/7
  Beta Lookup/2 -> Cld Elevon/6, CXd Elevon/6, Cmd Elevon/6, CYd Elevon/6, Cnd Elevon/6, CZd Elevon/6
  Beta Lookup/1 -> Cld Elevon/5, CXd Elevon/5, Cmd Elevon/5, CYd Elevon/5, Cnd Elevon/5, CZd Elevon/5
  Mach Lookup/2 -> Cnd Elevon/4, CZd Elevon/4, Cmd Elevon/4, CYd Elevon/4, CXd Elevon/4, Cld Elevon/4
  Mach Lookup/1 -> Cnd Elevon/3, CZd Elevon/3, Cmd Elevon/3, CYd Elevon/3, CXd Elevon/3, Cld Elevon/3
  Alpha Lookup/2 -> Cnd Elevon/2, CZd Elevon/2, Cmd Elevon/2, CYd Elevon/2, Cld Elevon/2, CXd Elevon/2
  Alpha Lookup/1 -> Cnd Elevon/1, CZd Elevon/1, Cmd Elevon/1, CYd Elevon/1, Cld Elevon/1, CXd Elevon/1
  albet/1 -> Demux/1
  Bus Selector1/1 -> Deltas Elevon/1  "<Elevon>"
  delta/1 -> Bus Selector1/1

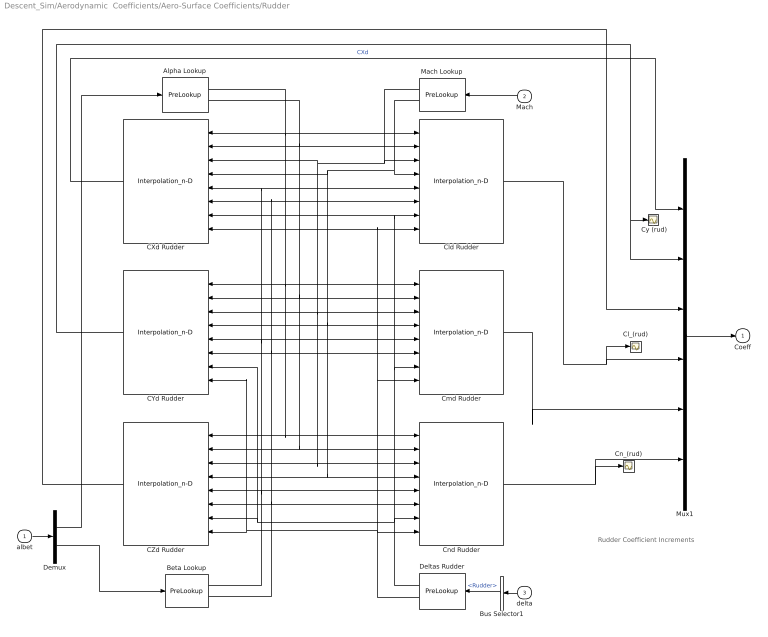
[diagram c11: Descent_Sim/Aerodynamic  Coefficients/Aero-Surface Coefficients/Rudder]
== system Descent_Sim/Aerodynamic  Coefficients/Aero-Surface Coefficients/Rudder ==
  note: Rudder Coefficient Increments
  albet : Inport  OutDataType=sfix(16)  OutScaling=2^0
  Mach : Inport  Port=2  OutDataType=sfix(16)  OutScaling=2^0
  delta : Inport  Port=3  OutDataType=sfix(16)  OutScaling=2^0
  " Cy (rud)" : Scope
  Alpha Lookup : PreLookup  BreakpointsData=Alfas  BeginIndexSearchUsingPreviousIndexResult=on  ProcessOutOfRangeInput=Linear extrapolation  IndexDataType=sfix(16)  FractionDataType=sfix(16)  FractionScaling=2^0
  Beta Lookup : PreLookup  BreakpointsData=Betas  BeginIndexSearchUsingPreviousIndexResult=on  ProcessOutOfRangeInput=Linear extrapolation  IndexDataType=sfix(16)  FractionDataType=sfix(16)  FractionScaling=2^0
  Bus Selector1 : BusSelector  OutputSignals=Rudder
  CXd Rudder : Interpolation_n-D  NumberOfTableDimensions=4  Table=CXd4  CheckIndexInCode=off  OutDataType=sfix(16)  OutScaling=2^0
  CYd Rudder : Interpolation_n-D  NumberOfTableDimensions=4  Table=CYd4  CheckIndexInCode=off  OutDataType=sfix(16)  OutScaling=2^0
  CZd Rudder : Interpolation_n-D  NumberOfTableDimensions=4  Table=CZd4  CheckIndexInCode=off  OutDataType=sfix(16)  OutScaling=2^0
  Cl_(rud) : Scope
  Cld Rudder : Interpolation_n-D  NumberOfTableDimensions=4  Table=Cld4  CheckIndexInCode=off  OutDataType=sfix(16)  OutScaling=2^0
  Cmd Rudder : Interpolation_n-D  NumberOfTableDimensions=4  Table=Cmd4  CheckIndexInCode=off  OutDataType=sfix(16)  OutScaling=2^0
  Cn_(rud) : Scope
  Cnd Rudder : Interpolation_n-D  NumberOfTableDimensions=4  Table=Cnd4  CheckIndexInCode=off  OutDataType=sfix(16)  OutScaling=2^0
  Deltas Rudder : PreLookup  BreakpointsData=Deltas4  BeginIndexSearchUsingPreviousIndexResult=on  ProcessOutOfRangeInput=Linear extrapolation  IndexDataType=sfix(16)  FractionDataType=sfix(16)  FractionScaling=2^0
  Demux : Demux  Outputs=2
  Mach Lookup : PreLookup  BreakpointsData=Machs  BeginIndexSearchUsingPreviousIndexResult=on  ProcessOutOfRangeInput=Linear extrapolation  IndexDataType=sfix(16)  FractionDataType=sfix(16)  FractionScaling=2^0
  Mux1 : Mux  Inputs=6
  Coeff : Outport  OutDataType=sfix(16)  OutScaling=2^0  InitialOutput=0
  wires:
  CZd Rudder/1 -> Mux1/3
  CYd Rudder/1 -> Mux1/2, " Cy (rud)"/1
  CXd Rudder/1 -> Mux1/1  "CXd"
  delta/1 -> Bus Selector1/1
  Demux/2 -> Beta Lookup/1
  Mach/1 -> Mach Lookup/1
  Demux/1 -> Alpha Lookup/1
  Cld Rudder/1 -> Mux1/4, Cl_(rud)/1
  Cmd Rudder/1 -> Mux1/5
  Cnd Rudder/1 -> Mux1/6, Cn_(rud)/1
  Mux1/1 -> Coeff/1
  Deltas Rudder/2 -> CXd Rudder/8, Cld Rudder/8, Cmd Rudder/8, Cnd Rudder/8, CYd Rudder/8, CZd Rudder/8
  Deltas Rudder/1 -> CXd Rudder/7, Cld Rudder/7, Cmd Rudder/7, Cnd Rudder/7, CYd Rudder/7, CZd Rudder/7
  Beta Lookup/2 -> Cld Rudder/6, CXd Rudder/6, Cmd Rudder/6, CYd Rudder/6, Cnd Rudder/6, CZd Rudder/6
  Beta Lookup/1 -> Cld Rudder/5, CXd Rudder/5, Cmd Rudder/5, CYd Rudder/5, Cnd Rudder/5, CZd Rudder/5
  Mach Lookup/2 -> Cnd Rudder/4, CZd Rudder/4, Cmd Rudder/4, CYd Rudder/4, CXd Rudder/4, Cld Rudder/4
  Mach Lookup/1 -> Cnd Rudder/3, CZd Rudder/3, Cmd Rudder/3, CYd Rudder/3, CXd Rudder/3, Cld Rudder/3
  Alpha Lookup/2 -> Cnd Rudder/2, CZd Rudder/2, Cmd Rudder/2, CYd Rudder/2, Cld Rudder/2, CXd Rudder/2
  Alpha Lookup/1 -> Cnd Rudder/1, CZd Rudder/1, Cmd Rudder/1, CYd Rudder/1, Cld Rudder/1, CXd Rudder/1
  albet/1 -> Demux/1
  Bus Selector1/1 -> Deltas Rudder/1  "<Rudder>"

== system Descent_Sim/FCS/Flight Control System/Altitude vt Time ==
  Demux : Demux  Tag=STV Demux  Outputs=1
  FromWs : FromWorkspace  Tag=STV FromWs  VariableName=tuvar  SampleTime=0  SigBuilderData=DataTag0  VnvData=DataTag1
  Signal 1 : Outport  Tag=STV Outport  OutDataType=fixdt(1, 16)  OutScaling=2^0
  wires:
  FromWs/1 -> Demux/1
  Demux/1 -> Signal 1/1
